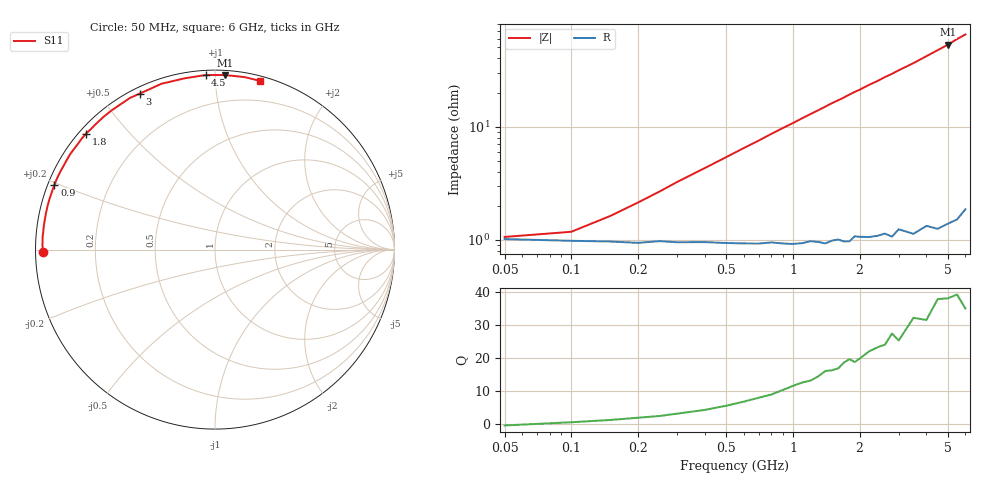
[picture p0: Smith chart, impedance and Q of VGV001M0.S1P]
! Infineon Technologies  Discrete & RF Semiconductors
! BB 831
! Si Tuning Diode in SOD323
! VR =
! S-Parameters:  July  1999
# GHz  S  MA  R  50
!  f  S11
! GHz  MAG  ANG
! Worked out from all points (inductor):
!   34 points, 50 MHz to 6 GHz, reference 50 ohm
!   read as one part to ground: L = 1.67 nH near 300 MHz
!   highest Q = 38 at 5 GHz (marker M1), where L = 1.68 nH
!   S11 on the Smith chart (normalised r, x): 50 MHz: 0.02, -0.01; 900 MHz: 0.02, +0.19; 1.8 GHz: 0.02, +0.38; 3 GHz: 0.02, +0.63; 4.5 GHz: 0.03, +0.95; 6 GHz: 0.04, +1.30
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0.05  0.9601 -179.3
0.1  0.9615 178.5
0.2  0.9631 175.6
0.3  0.9627 172.9
0.5  0.9636 167.9
0.6  0.964 165.4
0.7  0.9643 163.0
0.8  0.9638 160.5
0.9  0.9648 158.1
1.1  0.9652 153.4
1.4  0.9664 146.6
1.5  0.9649 144.3
1.6  0.9645 142.3
1.7  0.9663 140.2
1.8  0.9667 138.0
1.9  0.9637 135.9
2  0.9645 134.1
2.2  0.9658 130.0
2.4  0.966 126.5
2.6  0.9656 122.6
2.8  0.9687 119.3
3  0.9651 115.7
3.5  0.9709 107.9
4  0.9692 100.1
4.5  0.9739 93.1
5  0.9741 86.8
5.5  0.9752 80.2
6  0.9728 75.0
